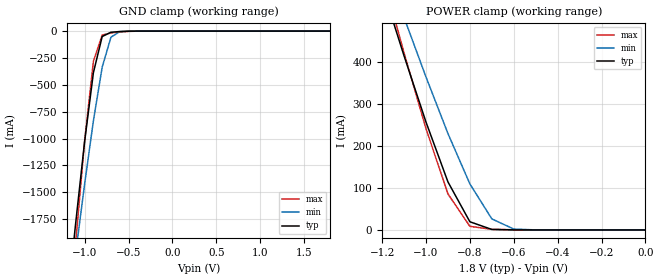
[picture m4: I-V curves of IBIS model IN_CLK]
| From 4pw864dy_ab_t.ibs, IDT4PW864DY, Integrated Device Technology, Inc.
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|   Model IN_CLK
[Model]   IN_CLK
Model_type   Input
Vinl =  0.37500V
Vinh =  1.42500V
C_comp   1.950000pF   1.950000pF   1.950000pF
[Temperature Range]   25.00000   0.11000k   0.000
[Voltage Range]   1.80000V   1.70000V   1.90000V
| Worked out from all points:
|   GND clamp passes 1 mA (typ) near -0.49 V on its own axis
|   POWER clamp passes 1 mA (typ) near -0.68 V on its own axis
[GND_clamp]
| voltage   I(typ)   I(min)   I(max)
-1.8V     -7.517A    -6.784A    -9.227A
-1.2V     -2.555A    -2.703A    -2.937A
-1.1V     -1.771A    -2.052A    -1.947A
-1V       -1.027A    -1.423A    -1.021A
-900mV    -386.6mA   -833.8mA   -281.6mA
-800mV    -50.87mA   -335.5mA   -36.73mA
-700mV    -10.76mA   -56.75mA   -17.58mA
-600mV    -4.165mA   -5.301mA   -8.844mA
-300mV    -18.14uA   -9.324uA   -72.3uA
1.8V      1.48nA     7.75nA     1.123nA
[POWER_clamp]
| voltage   I(typ)   I(min)   I(max)
-1.8V     1.609A     1.556A     1.801A
-1.2V     578.3mA    650.5mA    610.1mA
-1.1V     414mA      505.1mA    421mA
-1V       256.5mA    363.7mA    240.9mA
-900mV    114.3mA    229.3mA    85.69mA
-800mV    19.5mA     109.5mA    8.621mA
-700mV    1.233mA    26.32mA    1.539mA
-600mV    182.5uA    2.178mA    478.7uA
-500mV    28.06uA    143.3uA    93.54uA
0V        1.48nA     891pA      1.263nA
